(* Logix 5000 AddOnInstructionDefinition export AOI_Weber_C30S_EnIP_Mapper; software revision 20.01 *)

TYPE UDT_PLC2_to_30S :   // Output from PLC
STRUCT
   Automatic : BOOL;
   Start : BOOL;
   AckFault : BOOL;
   DS1 : BOOL;
   DS2 : BOOL;
   ExtDigSig : BOOL;
   Res1 : BOOL;
   Res2 : BOOL;
   Prog : SINT;
END_STRUCT
END_TYPE

TYPE UDT_C30S_to_PLC :   // Input to PLC
STRUCT
   NoFault : BOOL;
   ReadyToStart : BOOL;
   OK : BOOL;
   NOK : BOOL;
   DepthReached : BOOL;
   Res1 : BOOL;
   Res2 : BOOL;
   Res3 : BOOL;
   ProgResult : SINT;
   StrategyResult : SINT;
   CodeResult : INT;
   TorqueResult : REAL;
   PreTorqueResult : REAL;
   AngleResult : REAL;
   DepthResult : REAL;
   DriveTime : REAL;
   CycleNumber : DINT;
END_STRUCT
END_TYPE

TYPE UDT_C30S_EnIP :   // In and Output Data for Weber C30S
STRUCT
   OUT : UDT_PLC2_to_30S;   // Output Parameters
   IN : UDT_C30S_to_PLC;   // Input Parameters
END_STRUCT
END_TYPE

ADD_ON_INSTRUCTION AOI_Weber_C30S_EnIP_Mapper   (* revision 1.0, vendor Weber Schraubautomaten *)
// Maps Ethernet IO Data to UDT_C30S
// Revision note:
// 18/02/2014 Create
VAR_IN_OUT
   Screwdriver_Data : UDT_C30S_EnIP; {required}
   Field_Inputs : AB:ETHERNET_MODULE_SINT_29Bytes:I:0; {required}   // Inputs from Ethernet Module
   Field_Outputs : AB:ETHERNET_MODULE_SINT_2Bytes:O:0; {required}   // Outputs to Ethernet Module
END_VAR
VAR
   TempReal : REAL; {access None}
   TempDint : DINT; {access None}
END_VAR

ROUTINE Logic   (* ladder *)
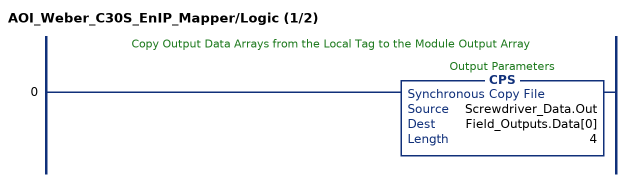
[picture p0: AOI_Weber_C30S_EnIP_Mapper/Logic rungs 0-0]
   // Copy Output Data Arrays from the Local Tag to the Module Output Array
   0: CPS(Screwdriver_Data.Out,Field_Outputs.Data[0],4);
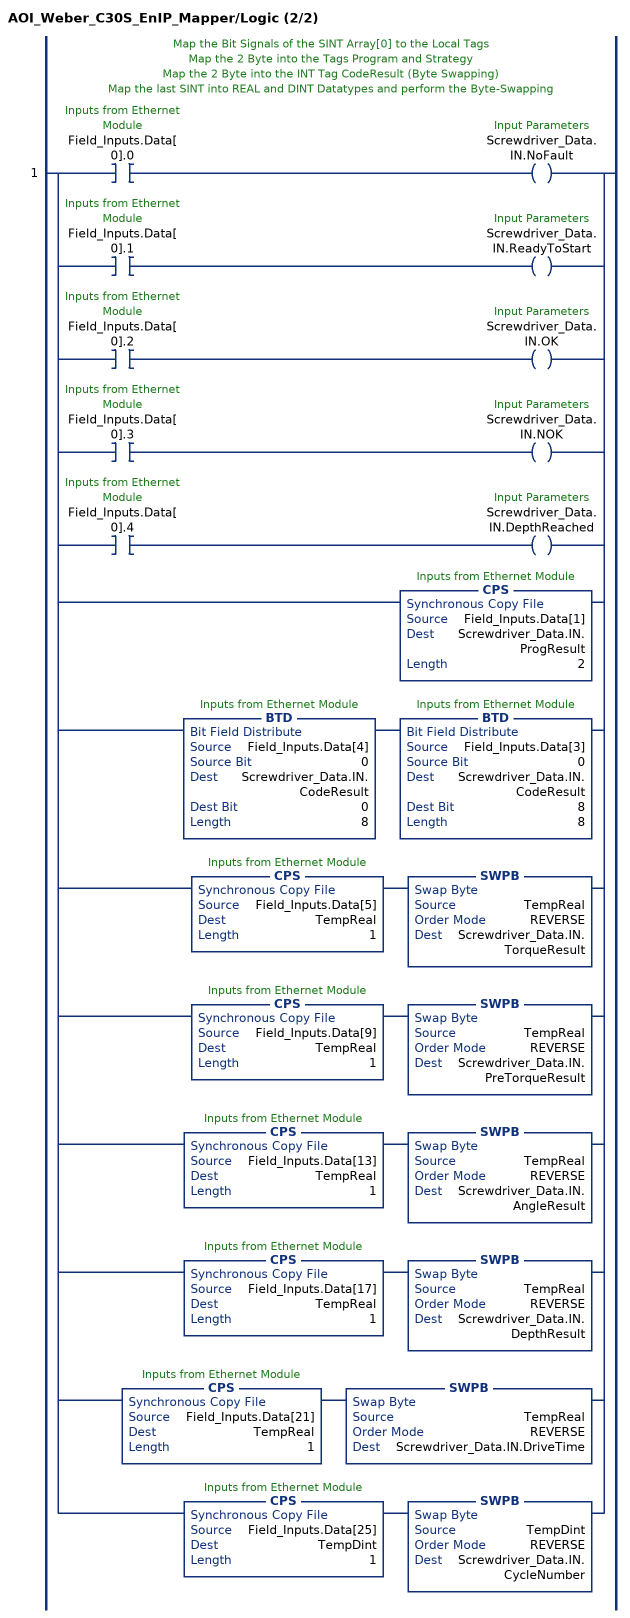
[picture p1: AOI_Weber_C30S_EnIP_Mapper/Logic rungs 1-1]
   // Map the Bit Signals of the SINT Array[0] to the Local Tags
   // Map the 2 Byte into the Tags Program and Strategy
   // Map the 2 Byte into the INT Tag CodeResult (Byte Swapping)
   // Map the last SINT into REAL and DINT Datatypes and perform the Byte-Swapping
   1: [XIC(Field_Inputs.Data[0].0) OTE(Screwdriver_Data.IN.NoFault) ,XIC(Field_Inputs.Data[0].1) OTE(Screwdriver_Data.IN.ReadyToStart) ,XIC(Field_Inputs.Data[0].2) OTE(Screwdriver_Data.IN.OK) ,XIC(Field_Inputs.Data[0].3) OTE(Screwdriver_Data.IN.NOK) ,XIC(Field_Inputs.Data[0].4) OTE(Screwdriver_Data.IN.DepthReached) ,CPS(Field_Inputs.Data[1],Screwdriver_Data.IN.ProgResult,2) ,BTD(Field_Inputs.Data[4],0,Screwdriver_Data.IN.CodeResult,0,8) BTD(Field_Inputs.Data[3],0,Screwdriver_Data.IN.CodeResult,8,8) ,CPS(Field_Inputs.Data[5],TempReal,1) SWPB(TempReal,REVERSE,Screwdriver_Data.IN.TorqueResult) ,CPS(Field_Inputs.Data[9],TempReal,1) SWPB(TempReal,REVERSE,Screwdriver_Data.IN.PreTorqueResult) ,CPS(Field_Inputs.Data[13],TempReal,1) SWPB(TempReal,REVERSE,Screwdriver_Data.IN.AngleResult) ,CPS(Field_Inputs.Data[17],TempReal,1) SWPB(TempReal,REVERSE,Screwdriver_Data.IN.DepthResult) ,CPS(Field_Inputs.Data[21],TempReal,1) SWPB(TempReal,REVERSE,Screwdriver_Data.IN.DriveTime) ,CPS(Field_Inputs.Data[25],TempDint,1) SWPB(TempDint,REVERSE,Screwdriver_Data.IN.CycleNumber) ];
END_ROUTINE
END_ADD_ON_INSTRUCTION
